FUNCTION_BLOCK FB19
TITLE =Set Position Regulation Gain
//*****************************************************************************
//* maxon motor ag
//* R&D
//* all rights reserved
//*****************************************************************************
//* Summary:  Set position regulation gains (PI)
//*
//* Remarks:
//*
//* Created under: STEP7 REV5.2+SP1
//*****************************************************************************
//* History:
//* 18.05.2004 | INA   first release
//*
//*
//*****************************************************************************
//

AUTHOR:INA
FAMILY:Configur
NAME:SPosRegG
VERSION:00.01


VAR_INPUT

Write : BOOL //A rising edge start the command

  NodeID : BYTE //Adress of the maxon device

  P_Gain : WORD //Position Regulator P-Gain

  I_Gain : WORD //Position Regulator I-Gain

  D_Gain : WORD //Position Regulator D-Gain

END_VAR
VAR_OUTPUT
  Done : BOOL //Data valid flag is TRUE if data were available

  Err : BOOL //Error flag is TRUE if an Error has occured, see ErrNo for more details

  ErrNo : DINT //Contains detailed error information

END_VAR
VAR
  xEdgeMerker : BOOL //Edge Merker

  xEdgeFlag : BOOL //Edge Flag

  xStep : INT
END_VAR

BEGIN

NETWORK
TITLE = Activate the service function
//

// SDO Write "Set Position Regulation Gain"

       U    #Write
       FP   #xEdgeFlag                   // recognize a positiv edge of the Read signal
       =    #xEdgeMerker                 // and set the xEdgeMerker for one cycle to true

       L    #xStep
       L    0
       ==I
       U    #xEdgeMerker
       SPB  nstp                         // iStep = 1 -> fnc1

       L    #xStep                       // jump list
       SPL  List
       SPA  rdef
       SPA  fnc1
       SPA  fncE
List  :SPA  rdef

rdef  :NOP  0
       R    #Done                        // reset Done
       R    #Err
       L    0
       T    #xStep                       // iStep = 0
       SPA  end

fnc1  :NOP  0
       CALL FC15
         NodeID:=#NodeID
         Index:=DW#16#000060FB
         SubIndex:=DW#16#00000001
         ValueIn:=#P_Gain
         RET_VAL:=#Done
         Err:=#Err
         ErrNo:=#ErrNo

       L    1
       U    #Err
       SPB  fncE

       NOP  0
       CALL FC15
         NodeID:=#NodeID
         Index:=DW#16#000060FB
         SubIndex:=DW#16#00000002
         ValueIn:=#I_Gain
         RET_VAL:=#Done
         Err:=#Err
         ErrNo:=#ErrNo

       L    1
       U    #Err
       SPB  fncE

       NOP  0
       CALL FC15
         NodeID:=#NodeID
         Index:=DW#16#000060FB
         SubIndex:=DW#16#00000003
         ValueIn:=#D_Gain
         RET_VAL:=#Done
         Err:=#Err
         ErrNo:=#ErrNo

fncE  :NOP  0
       L    0
       T    #xStep
       SPA  end

nstp  :NOP  0
       L    #xStep
       INC            1
       T    #xStep

end   :NOP  0
END_FUNCTION_BLOCK
